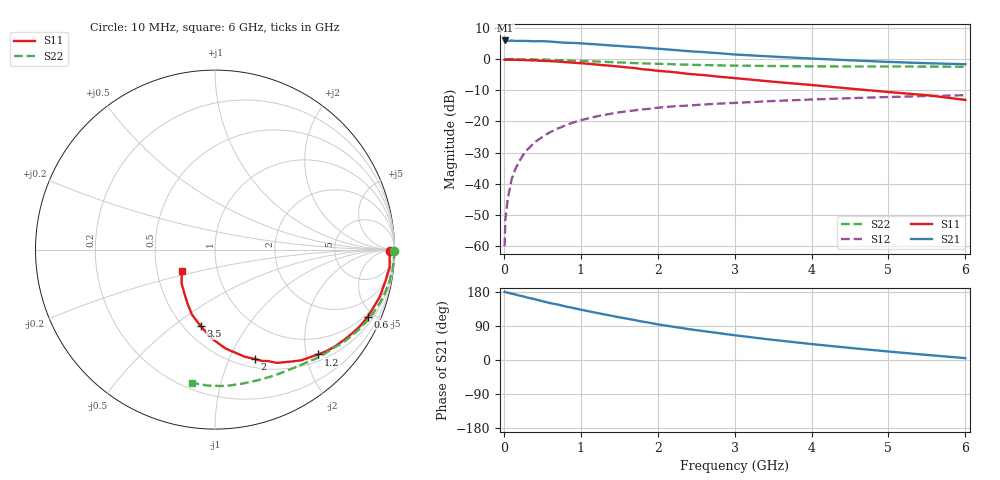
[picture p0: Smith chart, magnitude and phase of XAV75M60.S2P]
! SIEMENS Discrete & RF Semiconductors
! BFY180
! Si NPN RF Bipolar Junction Transistor in MICRO-X
! VCE = 0.75 V  IC = 0.6 mA
! Common Emitter S-Parameters:  May  1997
# GHz  S  MA  R  50
!  f  S11  S21  S12  S22
! GHz  MAG  ANG  MAG  ANG  MAG  ANG  MAG  ANG
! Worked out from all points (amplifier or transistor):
!   36 points, 10 MHz to 6 GHz, reference 50 ohm
!   highest |S21| = 6.0 dB at 20 MHz (marker M1)
!   |S21| within 3 dB of that: start of sweep to 2.184 GHz
!   unconditionally stable (mu >= 1): 3.745 GHz to end of sweep
!   at 250 MHz: K = 0.08, MSG = 18.3 dB, |S12| = -30.8 dB
!   at 1.4 GHz: K = 0.49, MSG = 10.9 dB, |S12| = -17.5 dB
!   at 6 GHz: K = 1.11, MAG = 3.0 dB, |S12| = -11.6 dB
!   S11 on the Smith chart (normalised r, x): 10 MHz: 77, -16; 600 MHz: 0.84, -4.62; 1.2 GHz: 0.63, -2.24; 2 GHz: 0.59, -1.25; 3.5 GHz: 0.60, -0.63; 6 GHz: 0.67, -0.17
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0.01  0.9756 -0.3  1.972 179.9  0.001 98.3  0.9979 -0.3
0.02  0.9741 -0.8  1.993 179.0  0.0027 96.3  0.9982 -0.5
0.05  0.9738 -1.9  1.954 177.8  0.0056 85.8  0.9965 -1.3
0.1  0.9755 -4.0  1.986 175.2  0.0117 88.8  0.9991 -2.7
0.15  0.9779 -6.1  1.959 172.9  0.0173 86.0  0.9992 -3.9
0.2  0.97 -8.0  1.96 170.2  0.023 84.2  0.9958 -5.2
0.3  0.9615 -12.1  1.954 165.1  0.0347 80.7  0.9908 -7.8
0.4  0.9551 -15.9  1.933 160.5  0.0463 78.2  0.9884 -10.4
0.6  0.9297 -23.7  1.912 150.2  0.0672 72.0  0.9753 -15.4
0.9  0.8776 -35.0  1.821 137.3  0.0962 63.1  0.9476 -22.5
1.1  0.8422 -42.0  1.757 128.7  0.1123 58.2  0.9264 -26.9
1.2  0.8194 -45.5  1.728 124.6  0.1202 55.4  0.9167 -29.2
1.5  0.7584 -55.2  1.626 112.7  0.1402 48.8  0.8844 -35.2
1.7  0.7192 -61.4  1.57 105.3  0.1507 45.0  0.8631 -38.7
2  0.6504 -69.8  1.471 94.1  0.1662 40.0  0.8418 -43.8
2.2  0.6199 -74.4  1.406 87.9  0.1746 36.6  0.8288 -47.1
2.4  0.5799 -79.7  1.341 81.6  0.1801 33.9  0.8123 -50.1
2.8  0.5224 -87.9  1.243 70.7  0.1934 29.0  0.7939 -55.7
3.5  0.4342 -100.5  1.098 53.1  0.213 21.7  0.7752 -65.1
4.5  0.337 -117.1  0.958 31.9  0.2363 12.1  0.7623 -78.7
5.5  0.2641 -134.9  0.86 13.4  0.256 2.9  0.7588 -92.9
6  0.2215 -146.6  0.828 4.9  0.2638 -1.8  0.7537 -99.9
